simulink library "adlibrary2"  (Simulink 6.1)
undefined symbols (not defined in the file or in its folder): adlibrary2, ADM, Bit, Black, Box, d2sram_config, DDR, ddr32_config, ddr32xp_config, Generation, II, Inactive, Location, Lower, SDRAM, Simulation, Subsystem, Width, xbsIndex_r3, XPL, XRC, XRM, zbt32_config, zbt64_config, zbtXRC4_config
libraries: xbsIndex_r3 x786
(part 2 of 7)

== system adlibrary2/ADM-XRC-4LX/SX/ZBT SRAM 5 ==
  d : Inport  Port=1  LatchInput=off
  a : Inport  Port=2  LatchInput=off
  w : Inport  Port=3  LatchInput=off
  r : Inport  Port=4  LatchInput=off
  be : Inport  Port=5  LatchInput=off
  adlocb_in : Inport  Port=6  LatchInput=off
  Constant : xbsIndex_r3/Constant  const=0  equ=P=C  arith_type=Unsigned  n_bits=34  bin_pt=0  opselect=C  inp2=PCIN>>17  opr=+  inp1=P  carry=CIN  iostate=0  explicit_period=on  period=1  dbl_ovrd=off
  Convert : xbsIndex_r3/Convert  arith_type=Unsigned  n_bits=34  bin_pt=0  quantization=Truncate  overflow=Wrap  latency=0  explicit_period=on  period=1  dbl_ovrd=off  show_param=off  inserted_by_tool=off  pipeline=off
  Simulation Multiplexer : xbsIndex_r3/Simulation Multiplexer  sim_sel=1  hw_sel=2
  Simulation Multiplexer1 : xbsIndex_r3/Simulation Multiplexer  sim_sel=1  hw_sel=2
  Simulation Multiplexer2 : xbsIndex_r3/Simulation Multiplexer  sim_sel=1  hw_sel=2
  ZBT SRAM 32Bit Generation : Subsystem
  ZBT SRAM 32Bit Simulation : Subsystem
  q : Outport
  qv : Outport  Port=2
  adlocb_out : Outport  Port=3
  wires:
  r/1 -> ZBT SRAM 32Bit Generation/4(r), ZBT SRAM 32Bit Simulation/4(r)
  w/1 -> ZBT SRAM 32Bit Generation/3(w), ZBT SRAM 32Bit Simulation/3(w)
  a/1 -> ZBT SRAM 32Bit Generation/2(a), ZBT SRAM 32Bit Simulation/2(a)
  d/1 -> ZBT SRAM 32Bit Generation/1(d), ZBT SRAM 32Bit Simulation/1(d)
  ZBT SRAM 32Bit Simulation/2(qv) -> Simulation Multiplexer1/1
  ZBT SRAM 32Bit Simulation/1(q) -> Simulation Multiplexer/1
  ZBT SRAM 32Bit Generation/1(q) -> Simulation Multiplexer/2
  ZBT SRAM 32Bit Generation/2(qv) -> Simulation Multiplexer1/2
  Simulation Multiplexer1/1 -> qv/1
  Simulation Multiplexer/1 -> q/1
  be/1 -> ZBT SRAM 32Bit Simulation/5(be), ZBT SRAM 32Bit Generation/5(be)
  Simulation Multiplexer2/1 -> adlocb_out/1
  ZBT SRAM 32Bit Generation/3(adlocb_out) -> Convert/1
  adlocb_in/1 -> ZBT SRAM 32Bit Generation/6(adlocb_in)
  Constant/1 -> Simulation Multiplexer2/1
  Convert/1 -> Simulation Multiplexer2/2

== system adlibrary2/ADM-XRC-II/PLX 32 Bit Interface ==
  Data_Read : Inport  Port=1  LatchInput=off
  Ack : Inport  Port=2  LatchInput=off
  Status : Inport  Port=3  LatchInput=off
  Read IFIFO : Inport  Port=4  LatchInput=off
  Write OFIFO : Inport  Port=5  LatchInput=off
  OFIFO_Data : Inport  Port=6  LatchInput=off
  ADLOCB_IN : Inport  Port=7  LatchInput=off
  Constant : xbsIndex_r3/Constant  const=0  equ=P=C  arith_type=Unsigned  n_bits=34  bin_pt=0  opselect=C  inp2=PCIN>>17  opr=+  inp1=P  carry=CIN  iostate=0  explicit_period=on  period=1  dbl_ovrd=off
  Convert : xbsIndex_r3/Convert  arith_type=Unsigned  n_bits=34  bin_pt=0  quantization=Truncate  overflow=Wrap  latency=0  explicit_period=on  period=1  dbl_ovrd=off  show_param=off  inserted_by_tool=off  pipeline=off
  PLX 32Bit Generation : Subsystem
  PLX 32Bit Simulation : Subsystem  mask{program=program, clock_ratio=clock_ratio}
      mask prompts: program "Local Bus Script Program"; clock_ratio "Clock Ratio"
  Simulation Multiplexer{,1..9} (10 alike) : xbsIndex_r3/Simulation Multiplexer  sim_sel=1  hw_sel=2
  Data_Write : Outport
  Addr : Outport  Port=2
  BE : Outport  Port=3
  Write : Outport  Port=4
  Read : Outport  Port=5
  Control : Outport  Port=6
  IFIFO_Data : Outport  Port=7
  IFIFO_Empty : Outport  Port=8
  OFIFO_Full : Outport  Port=9
  ADLOCB_OUT : Outport  Port=10
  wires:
  Data_Read/1 -> PLX 32Bit Generation/1(Data_Read), PLX 32Bit Simulation/1(Data_Read)
  Ack/1 -> PLX 32Bit Generation/2(Ack), PLX 32Bit Simulation/2(Ack)
  Status/1 -> PLX 32Bit Generation/3(Status), PLX 32Bit Simulation/3(Status)
  Read IFIFO/1 -> PLX 32Bit Generation/4(Read IFIFO), PLX 32Bit Simulation/4(Read IFIFO)
  Write OFIFO/1 -> PLX 32Bit Generation/5(Write OFIFO), PLX 32Bit Simulation/5(Write OFIFO)
  OFIFO_Data/1 -> PLX 32Bit Generation/6(OFIFO_Data), PLX 32Bit Simulation/6(OFIFO_Data)
  Simulation Multiplexer/1 -> Data_Write/1
  Simulation Multiplexer1/1 -> Addr/1
  Simulation Multiplexer2/1 -> Write/1
  Simulation Multiplexer3/1 -> Read/1
  Simulation Multiplexer4/1 -> Control/1
  Simulation Multiplexer5/1 -> IFIFO_Data/1
  Simulation Multiplexer6/1 -> IFIFO_Empty/1
  Simulation Multiplexer7/1 -> OFIFO_Full/1
  PLX 32Bit Generation/9(OFIFO_Full) -> Simulation Multiplexer7/2
  PLX 32Bit Generation/8(IFIFO_Empty) -> Simulation Multiplexer6/2
  PLX 32Bit Generation/7(IFIFO_Data) -> Simulation Multiplexer5/2
  PLX 32Bit Generation/6(Control) -> Simulation Multiplexer4/2
  PLX 32Bit Generation/5(Read) -> Simulation Multiplexer3/2
  PLX 32Bit Generation/4(Write) -> Simulation Multiplexer2/2
  PLX 32Bit Generation/2(Addr) -> Simulation Multiplexer1/2
  PLX 32Bit Generation/1(Data_Write) -> Simulation Multiplexer/2
  PLX 32Bit Simulation/1(Data_Write) -> Simulation Multiplexer/1
  PLX 32Bit Simulation/2(Addr) -> Simulation Multiplexer1/1
  PLX 32Bit Simulation/4(Write) -> Simulation Multiplexer2/1
  PLX 32Bit Simulation/5(Read) -> Simulation Multiplexer3/1
  PLX 32Bit Simulation/6(Control) -> Simulation Multiplexer4/1
  PLX 32Bit Simulation/7(IFIFO_Data) -> Simulation Multiplexer5/1
  PLX 32Bit Simulation/8(IFIFO_Empty) -> Simulation Multiplexer6/1
  PLX 32Bit Simulation/9(OFIFO_Full) -> Simulation Multiplexer7/1
  Simulation Multiplexer8/1 -> BE/1
  PLX 32Bit Generation/3(BE) -> Simulation Multiplexer8/2
  PLX 32Bit Simulation/3(BE) -> Simulation Multiplexer8/1
  Simulation Multiplexer9/1 -> ADLOCB_OUT/1
  PLX 32Bit Generation/10(ADLOCB_OUT) -> Convert/1
  ADLOCB_IN/1 -> PLX 32Bit Generation/7(ADLOCB_IN)
  Constant/1 -> Simulation Multiplexer9/1
  Convert/1 -> Simulation Multiplexer9/2

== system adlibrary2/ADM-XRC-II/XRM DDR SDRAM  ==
  cache_data_in : Inport  Port=1  LatchInput=off
  cache_addr : Inport  Port=2  LatchInput=off
  cache_write : Inport  Port=3  LatchInput=off
  ddr_page : Inport  Port=4  LatchInput=off
  ddr_addr : Inport  Port=5  LatchInput=off
  ddr_read : Inport  Port=6  LatchInput=off
  ddr_write : Inport  Port=7  LatchInput=off
  DDR SDRAM 64Bit Generation : Subsystem
  DDR SDRAM 64bit Simulation : Subsystem  mask{memsize=memsize}
      mask prompts: memsize "Simulation Ram Size (Mb)"
  Simulation Multiplexer : xbsIndex_r3/Simulation Multiplexer  sim_sel=1  hw_sel=2
  Simulation Multiplexer1 : xbsIndex_r3/Simulation Multiplexer  sim_sel=1  hw_sel=2
  Terminator1 : Terminator
  cache_data_out : Outport
  ddr_busy : Outport  Port=2
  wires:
  cache_data_in/1 -> DDR SDRAM 64bit Simulation/1(cache_data_in), DDR SDRAM 64Bit Generation/1(cache_data_in)
  cache_addr/1 -> DDR SDRAM 64bit Simulation/2(cache_addr), DDR SDRAM 64Bit Generation/2(cache_addr)
  cache_write/1 -> DDR SDRAM 64bit Simulation/3(cache_write), DDR SDRAM 64Bit Generation/3(cache_write)
  ddr_page/1 -> DDR SDRAM 64bit Simulation/4(ddr_page), DDR SDRAM 64Bit Generation/4(ddr_page)
  ddr_addr/1 -> DDR SDRAM 64bit Simulation/5(ddr_addr), DDR SDRAM 64Bit Generation/5(ddr_addr)
  ddr_read/1 -> DDR SDRAM 64Bit Generation/6(ddr_read), DDR SDRAM 64bit Simulation/6(ddr_read)
  ddr_write/1 -> DDR SDRAM 64Bit Generation/7(ddr_write), DDR SDRAM 64bit Simulation/7(ddr_write)
  Simulation Multiplexer/1 -> cache_data_out/1
  Simulation Multiplexer1/1 -> ddr_busy/1
  DDR SDRAM 64bit Simulation/3(ddr_status) -> Terminator1/1
  DDR SDRAM 64bit Simulation/2(ddr_busy) -> Simulation Multiplexer1/1
  DDR SDRAM 64bit Simulation/1(cache_data_out) -> Simulation Multiplexer/1
  DDR SDRAM 64Bit Generation/1(cache_data_out) -> Simulation Multiplexer/2
  DDR SDRAM 64Bit Generation/2(ddr_busy) -> Simulation Multiplexer1/2

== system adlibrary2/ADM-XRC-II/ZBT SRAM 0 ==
  d : Inport  Port=1  LatchInput=off
  a : Inport  Port=2  LatchInput=off
  w : Inport  Port=3  LatchInput=off
  r : Inport  Port=4  LatchInput=off
  be : Inport  Port=5  LatchInput=off
  adlocb_in : Inport  Port=6  LatchInput=off
  Constant : xbsIndex_r3/Constant  const=0  equ=P=C  arith_type=Unsigned  n_bits=34  bin_pt=0  opselect=C  inp2=PCIN>>17  opr=+  inp1=P  carry=CIN  iostate=0  explicit_period=on  period=1  dbl_ovrd=off
  Simulation Multiplexer : xbsIndex_r3/Simulation Multiplexer  sim_sel=1  hw_sel=2
  Simulation Multiplexer1 : xbsIndex_r3/Simulation Multiplexer  sim_sel=1  hw_sel=2
  Simulation Multiplexer2 : xbsIndex_r3/Simulation Multiplexer  sim_sel=1  hw_sel=2
  ZBT SRAM 32Bit Generation : Subsystem
  ZBT SRAM 32Bit Simulation : Subsystem
  q : Outport
  qv : Outport  Port=2
  adlocb_out : Outport  Port=3
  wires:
  r/1 -> ZBT SRAM 32Bit Generation/4(r), ZBT SRAM 32Bit Simulation/4(r)
  w/1 -> ZBT SRAM 32Bit Generation/3(w), ZBT SRAM 32Bit Simulation/3(w)
  a/1 -> ZBT SRAM 32Bit Generation/2(a), ZBT SRAM 32Bit Simulation/2(a)
  d/1 -> ZBT SRAM 32Bit Generation/1(d), ZBT SRAM 32Bit Simulation/1(d)
  ZBT SRAM 32Bit Simulation/2(qv) -> Simulation Multiplexer1/1
  ZBT SRAM 32Bit Simulation/1(q) -> Simulation Multiplexer/1
  ZBT SRAM 32Bit Generation/1(q) -> Simulation Multiplexer/2
  ZBT SRAM 32Bit Generation/2(qv) -> Simulation Multiplexer1/2
  Simulation Multiplexer1/1 -> qv/1
  Simulation Multiplexer/1 -> q/1
  be/1 -> ZBT SRAM 32Bit Simulation/5(be), ZBT SRAM 32Bit Generation/5(be)
  Simulation Multiplexer2/1 -> adlocb_out/1
  ZBT SRAM 32Bit Generation/3(adlocb_out) -> Simulation Multiplexer2/2
  adlocb_in/1 -> ZBT SRAM 32Bit Generation/6(adlocb_in)
  Constant/1 -> Simulation Multiplexer2/1

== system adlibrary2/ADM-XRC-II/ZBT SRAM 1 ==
  d : Inport  Port=1  LatchInput=off
  a : Inport  Port=2  LatchInput=off
  w : Inport  Port=3  LatchInput=off
  r : Inport  Port=4  LatchInput=off
  be : Inport  Port=5  LatchInput=off
  adlocb_in : Inport  Port=6  LatchInput=off
  Constant : xbsIndex_r3/Constant  const=0  equ=P=C  arith_type=Unsigned  n_bits=34  bin_pt=0  opselect=C  inp2=PCIN>>17  opr=+  inp1=P  carry=CIN  iostate=0  explicit_period=on  period=1  dbl_ovrd=off
  Convert : xbsIndex_r3/Convert  arith_type=Unsigned  n_bits=34  bin_pt=0  quantization=Truncate  overflow=Wrap  latency=0  explicit_period=on  period=1  dbl_ovrd=off  show_param=off  inserted_by_tool=off  pipeline=off
  Simulation Multiplexer : xbsIndex_r3/Simulation Multiplexer  sim_sel=1  hw_sel=2
  Simulation Multiplexer1 : xbsIndex_r3/Simulation Multiplexer  sim_sel=1  hw_sel=2
  Simulation Multiplexer2 : xbsIndex_r3/Simulation Multiplexer  sim_sel=1  hw_sel=2
  ZBT SRAM 32Bit Generation : Subsystem
  ZBT SRAM 32Bit Simulation : Subsystem
  q : Outport
  qv : Outport  Port=2
  adlocb_out : Outport  Port=3
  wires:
  Constant/1 -> Simulation Multiplexer2/1
  adlocb_in/1 -> ZBT SRAM 32Bit Generation/6(adlocb_in)
  ZBT SRAM 32Bit Generation/3(adlocb_out) -> Convert/1
  Simulation Multiplexer2/1 -> adlocb_out/1
  be/1 -> ZBT SRAM 32Bit Generation/5(be), ZBT SRAM 32Bit Simulation/5(be)
  Simulation Multiplexer/1 -> q/1
  Simulation Multiplexer1/1 -> qv/1
  ZBT SRAM 32Bit Generation/2(qv) -> Simulation Multiplexer1/2
  ZBT SRAM 32Bit Generation/1(q) -> Simulation Multiplexer/2
  ZBT SRAM 32Bit Simulation/1(q) -> Simulation Multiplexer/1
  ZBT SRAM 32Bit Simulation/2(qv) -> Simulation Multiplexer1/1
  d/1 -> ZBT SRAM 32Bit Simulation/1(d), ZBT SRAM 32Bit Generation/1(d)
  a/1 -> ZBT SRAM 32Bit Simulation/2(a), ZBT SRAM 32Bit Generation/2(a)
  w/1 -> ZBT SRAM 32Bit Simulation/3(w), ZBT SRAM 32Bit Generation/3(w)
  r/1 -> ZBT SRAM 32Bit Simulation/4(r), ZBT SRAM 32Bit Generation/4(r)
  Convert/1 -> Simulation Multiplexer2/2

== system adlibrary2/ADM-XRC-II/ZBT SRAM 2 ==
  d : Inport  Port=1  LatchInput=off
  a : Inport  Port=2  LatchInput=off
  w : Inport  Port=3  LatchInput=off
  r : Inport  Port=4  LatchInput=off
  be : Inport  Port=5  LatchInput=off
  adlocb_in : Inport  Port=6  LatchInput=off
  Constant : xbsIndex_r3/Constant  const=0  equ=P=C  arith_type=Unsigned  n_bits=34  bin_pt=0  opselect=C  inp2=PCIN>>17  opr=+  inp1=P  carry=CIN  iostate=0  explicit_period=on  period=1  dbl_ovrd=off
  Convert : xbsIndex_r3/Convert  arith_type=Unsigned  n_bits=34  bin_pt=0  quantization=Truncate  overflow=Wrap  latency=0  explicit_period=on  period=1  dbl_ovrd=off  show_param=off  inserted_by_tool=off  pipeline=off
  Simulation Multiplexer : xbsIndex_r3/Simulation Multiplexer  sim_sel=1  hw_sel=2
  Simulation Multiplexer1 : xbsIndex_r3/Simulation Multiplexer  sim_sel=1  hw_sel=2
  Simulation Multiplexer2 : xbsIndex_r3/Simulation Multiplexer  sim_sel=1  hw_sel=2
  ZBT SRAM 32Bit Generation : Subsystem
  ZBT SRAM 32Bit Simulation : Subsystem
  q : Outport
  qv : Outport  Port=2
  adlocb_out : Outport  Port=3
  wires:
  Constant/1 -> Simulation Multiplexer2/1
  adlocb_in/1 -> ZBT SRAM 32Bit Generation/6(adlocb_in)
  ZBT SRAM 32Bit Generation/3(adlocb_out) -> Convert/1
  Simulation Multiplexer2/1 -> adlocb_out/1
  be/1 -> ZBT SRAM 32Bit Generation/5(be), ZBT SRAM 32Bit Simulation/5(be)
  Simulation Multiplexer/1 -> q/1
  Simulation Multiplexer1/1 -> qv/1
  ZBT SRAM 32Bit Generation/2(qv) -> Simulation Multiplexer1/2
  ZBT SRAM 32Bit Generation/1(q) -> Simulation Multiplexer/2
  ZBT SRAM 32Bit Simulation/1(q) -> Simulation Multiplexer/1
  ZBT SRAM 32Bit Simulation/2(qv) -> Simulation Multiplexer1/1
  d/1 -> ZBT SRAM 32Bit Simulation/1(d), ZBT SRAM 32Bit Generation/1(d)
  a/1 -> ZBT SRAM 32Bit Simulation/2(a), ZBT SRAM 32Bit Generation/2(a)
  w/1 -> ZBT SRAM 32Bit Simulation/3(w), ZBT SRAM 32Bit Generation/3(w)
  r/1 -> ZBT SRAM 32Bit Simulation/4(r), ZBT SRAM 32Bit Generation/4(r)
  Convert/1 -> Simulation Multiplexer2/2

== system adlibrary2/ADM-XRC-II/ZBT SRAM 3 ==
  d : Inport  Port=1  LatchInput=off
  a : Inport  Port=2  LatchInput=off
  w : Inport  Port=3  LatchInput=off
  r : Inport  Port=4  LatchInput=off
  be : Inport  Port=5  LatchInput=off
  adlocb_in : Inport  Port=6  LatchInput=off
  Constant : xbsIndex_r3/Constant  const=0  equ=P=C  arith_type=Unsigned  n_bits=34  bin_pt=0  opselect=C  inp2=PCIN>>17  opr=+  inp1=P  carry=CIN  iostate=0  explicit_period=on  period=1  dbl_ovrd=off
  Convert : xbsIndex_r3/Convert  arith_type=Unsigned  n_bits=34  bin_pt=0  quantization=Truncate  overflow=Wrap  latency=0  explicit_period=on  period=1  dbl_ovrd=off  show_param=off  inserted_by_tool=off  pipeline=off
  Simulation Multiplexer : xbsIndex_r3/Simulation Multiplexer  sim_sel=1  hw_sel=2
  Simulation Multiplexer1 : xbsIndex_r3/Simulation Multiplexer  sim_sel=1  hw_sel=2
  Simulation Multiplexer2 : xbsIndex_r3/Simulation Multiplexer  sim_sel=1  hw_sel=2
  ZBT SRAM 32Bit Generation : Subsystem
  ZBT SRAM 32Bit Simulation : Subsystem
  q : Outport
  qv : Outport  Port=2
  adlocb_out : Outport  Port=3
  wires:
  r/1 -> ZBT SRAM 32Bit Generation/4(r), ZBT SRAM 32Bit Simulation/4(r)
  w/1 -> ZBT SRAM 32Bit Generation/3(w), ZBT SRAM 32Bit Simulation/3(w)
  a/1 -> ZBT SRAM 32Bit Generation/2(a), ZBT SRAM 32Bit Simulation/2(a)
  d/1 -> ZBT SRAM 32Bit Generation/1(d), ZBT SRAM 32Bit Simulation/1(d)
  ZBT SRAM 32Bit Simulation/2(qv) -> Simulation Multiplexer1/1
  ZBT SRAM 32Bit Simulation/1(q) -> Simulation Multiplexer/1
  ZBT SRAM 32Bit Generation/1(q) -> Simulation Multiplexer/2
  ZBT SRAM 32Bit Generation/2(qv) -> Simulation Multiplexer1/2
  Simulation Multiplexer1/1 -> qv/1
  Simulation Multiplexer/1 -> q/1
  be/1 -> ZBT SRAM 32Bit Simulation/5(be), ZBT SRAM 32Bit Generation/5(be)
  Simulation Multiplexer2/1 -> adlocb_out/1
  ZBT SRAM 32Bit Generation/3(adlocb_out) -> Convert/1
  adlocb_in/1 -> ZBT SRAM 32Bit Generation/6(adlocb_in)
  Constant/1 -> Simulation Multiplexer2/1
  Convert/1 -> Simulation Multiplexer2/2

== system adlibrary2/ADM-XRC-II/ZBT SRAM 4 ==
  d : Inport  Port=1  LatchInput=off
  a : Inport  Port=2  LatchInput=off
  w : Inport  Port=3  LatchInput=off
  r : Inport  Port=4  LatchInput=off
  be : Inport  Port=5  LatchInput=off
  adlocb_in : Inport  Port=6  LatchInput=off
  Constant : xbsIndex_r3/Constant  const=0  equ=P=C  arith_type=Unsigned  n_bits=34  bin_pt=0  opselect=C  inp2=PCIN>>17  opr=+  inp1=P  carry=CIN  iostate=0  explicit_period=on  period=1  dbl_ovrd=off
  Convert : xbsIndex_r3/Convert  arith_type=Unsigned  n_bits=34  bin_pt=0  quantization=Truncate  overflow=Wrap  latency=0  explicit_period=on  period=1  dbl_ovrd=off  show_param=off  inserted_by_tool=off  pipeline=off
  Simulation Multiplexer : xbsIndex_r3/Simulation Multiplexer  sim_sel=1  hw_sel=2
  Simulation Multiplexer1 : xbsIndex_r3/Simulation Multiplexer  sim_sel=1  hw_sel=2
  Simulation Multiplexer2 : xbsIndex_r3/Simulation Multiplexer  sim_sel=1  hw_sel=2
  ZBT SRAM 32Bit Generation : Subsystem
  ZBT SRAM 32Bit Simulation : Subsystem
  q : Outport
  qv : Outport  Port=2
  adlocb_out : Outport  Port=3
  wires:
  Constant/1 -> Simulation Multiplexer2/1
  adlocb_in/1 -> ZBT SRAM 32Bit Generation/6(adlocb_in)
  ZBT SRAM 32Bit Generation/3(adlocb_out) -> Convert/1
  Simulation Multiplexer2/1 -> adlocb_out/1
  be/1 -> ZBT SRAM 32Bit Generation/5(be), ZBT SRAM 32Bit Simulation/5(be)
  Simulation Multiplexer/1 -> q/1
  Simulation Multiplexer1/1 -> qv/1
  ZBT SRAM 32Bit Generation/2(qv) -> Simulation Multiplexer1/2
  ZBT SRAM 32Bit Generation/1(q) -> Simulation Multiplexer/2
  ZBT SRAM 32Bit Simulation/1(q) -> Simulation Multiplexer/1
  ZBT SRAM 32Bit Simulation/2(qv) -> Simulation Multiplexer1/1
  d/1 -> ZBT SRAM 32Bit Simulation/1(d), ZBT SRAM 32Bit Generation/1(d)
  a/1 -> ZBT SRAM 32Bit Simulation/2(a), ZBT SRAM 32Bit Generation/2(a)
  w/1 -> ZBT SRAM 32Bit Simulation/3(w), ZBT SRAM 32Bit Generation/3(w)
  r/1 -> ZBT SRAM 32Bit Simulation/4(r), ZBT SRAM 32Bit Generation/4(r)
  Convert/1 -> Simulation Multiplexer2/2

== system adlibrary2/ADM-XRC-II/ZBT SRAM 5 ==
  d : Inport  Port=1  LatchInput=off
  a : Inport  Port=2  LatchInput=off
  w : Inport  Port=3  LatchInput=off
  r : Inport  Port=4  LatchInput=off
  be : Inport  Port=5  LatchInput=off
  adlocb_in : Inport  Port=6  LatchInput=off
  Constant : xbsIndex_r3/Constant  const=0  equ=P=C  arith_type=Unsigned  n_bits=34  bin_pt=0  opselect=C  inp2=PCIN>>17  opr=+  inp1=P  carry=CIN  iostate=0  explicit_period=on  period=1  dbl_ovrd=off
  Convert : xbsIndex_r3/Convert  arith_type=Unsigned  n_bits=34  bin_pt=0  quantization=Truncate  overflow=Wrap  latency=0  explicit_period=on  period=1  dbl_ovrd=off  show_param=off  inserted_by_tool=off  pipeline=off
  Simulation Multiplexer : xbsIndex_r3/Simulation Multiplexer  sim_sel=1  hw_sel=2
  Simulation Multiplexer1 : xbsIndex_r3/Simulation Multiplexer  sim_sel=1  hw_sel=2
  Simulation Multiplexer2 : xbsIndex_r3/Simulation Multiplexer  sim_sel=1  hw_sel=2
  ZBT SRAM 32Bit Generation : Subsystem
  ZBT SRAM 32Bit Simulation : Subsystem
  q : Outport
  qv : Outport  Port=2
  adlocb_out : Outport  Port=3
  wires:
  r/1 -> ZBT SRAM 32Bit Generation/4(r), ZBT SRAM 32Bit Simulation/4(r)
  w/1 -> ZBT SRAM 32Bit Generation/3(w), ZBT SRAM 32Bit Simulation/3(w)
  a/1 -> ZBT SRAM 32Bit Generation/2(a), ZBT SRAM 32Bit Simulation/2(a)
  d/1 -> ZBT SRAM 32Bit Generation/1(d), ZBT SRAM 32Bit Simulation/1(d)
  ZBT SRAM 32Bit Simulation/2(qv) -> Simulation Multiplexer1/1
  ZBT SRAM 32Bit Simulation/1(q) -> Simulation Multiplexer/1
  ZBT SRAM 32Bit Generation/1(q) -> Simulation Multiplexer/2
  ZBT SRAM 32Bit Generation/2(qv) -> Simulation Multiplexer1/2
  Simulation Multiplexer1/1 -> qv/1
  Simulation Multiplexer/1 -> q/1
  be/1 -> ZBT SRAM 32Bit Simulation/5(be), ZBT SRAM 32Bit Generation/5(be)
  Simulation Multiplexer2/1 -> adlocb_out/1
  ZBT SRAM 32Bit Generation/3(adlocb_out) -> Convert/1
  adlocb_in/1 -> ZBT SRAM 32Bit Generation/6(adlocb_in)
  Constant/1 -> Simulation Multiplexer2/1
  Convert/1 -> Simulation Multiplexer2/2

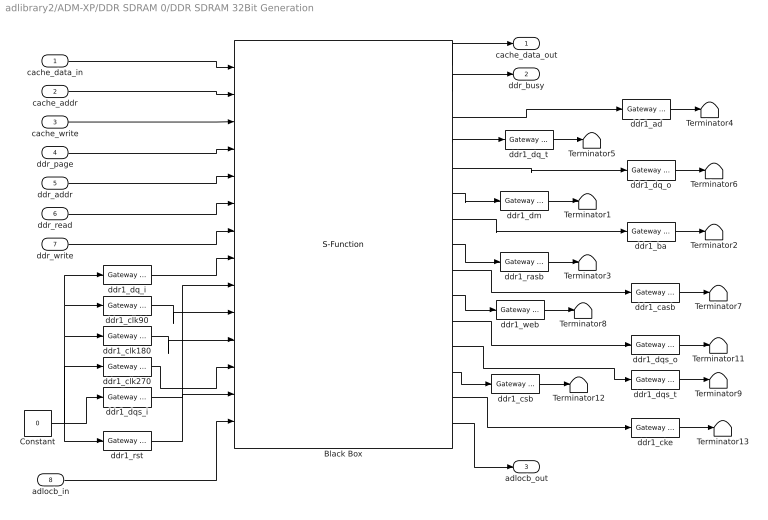
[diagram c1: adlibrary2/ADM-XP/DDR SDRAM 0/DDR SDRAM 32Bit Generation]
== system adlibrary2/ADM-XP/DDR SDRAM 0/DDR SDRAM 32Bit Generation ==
  cache_data_in : Inport  Port=1  LatchInput=off
  cache_addr : Inport  Port=2  LatchInput=off
  cache_write : Inport  Port=3  LatchInput=off
  ddr_page : Inport  Port=4  LatchInput=off
  ddr_addr : Inport  Port=5  LatchInput=off
  ddr_read : Inport  Port=6  LatchInput=off
  ddr_write : Inport  Port=7  LatchInput=off
  adlocb_in : Inport  Port=8  LatchInput=off
  Black Box : S-Function  AncestorBlock=xbsIndex_r3/Black Box  FunctionName=xlblackbox2  Parameters=sfcn_mwsv__  mask(Xilinx Blackbox Block){init_code=ddr32xp_config, sim_method=Inactive, engine_block=, show_param=on, xl_area=[375, 550, 2, 337, 9, 0, 0], xl_use_area=on, adlocb_devid=4, ddr_size=64}
      mask prompts: init_code "Block Configuration M-Function"; sim_method "Simulation Mode"; engine_block "HDL Co-Simulator To Use  (specify helper block by name)"; show_param "---------------------- Show Implementation Parameters -----------------------------------------------------------------------------------"; xl_area "FPGA Area [Slices, FFs, BRAMs, LUTs, IOBs, Emb. Mults, TBUFs]"; xl_use_area "Use Area Above For Estimation"; adlocb_devid "ADLOCB DEV ID"; ddr_size "DDR BANK SIZE(MB)"
      mask help: Incorporates black box HDL and simulation model into a System Generator design. You must supply a Black Box with certain information about the HDL component you would like to bring into System Generator. This information is provided through a Matlab function. When "Simulation Mode" is set to "Inactive," you will typically want to provide a separate simulation model by using a Simulation Multiplexer. When "Simulation Mode" is set to "Use HDL Co-Simulation", you must include a ModelSim block in the design.
      mask init:
      | [designRoot, family, part, speed, package, simulinkPeriod, sysclkPeriod, dbl_ovrd, trimVbit] = xlSysgenSettings(gcb,0,0);
      | 
      | [bg,fg] = xlcmap('XBlock');
      | iPos = get_param(gcb,'Position');
      | iWidth=iPos(3)-iPos(1); iHeight=iPos(4)-iPos(2);
      | iCx=iWidth/2;
      | iCy=iHeight/2;
      | [logoX, logoY] = xlogo(iPos);
      | zstr='z'; zpstr='-1';
      | zstrx = iCx-3; if (zstrx<16) zstr='';zpstr=''; end
      | zstry = iCy;
      | 
      | precision0 = 1;
      | latency = 0;
      | dblOvrd = 0;
      | 
      | mdlPath = xlGetMdlDir(bdroot);
      | 
      | refBlk = get_param(gcb,'referenceBlock');
      | if (isempty(refBlk) | strncmp(refBlk,'xbsIndex',8))
      | 	srcPath = mdlPath;
      | else
      | 	srcPath = xlPathToReference;
      | 	if (isempty(srcPath))
      | 		srcPath = mdlPath;
      | 	end
      | end
      | 
      | if (sim_method==2)
      | 	validEngineBlock = 0;
      | 	try
      | 	  engineBlock = xlBlockNameRelPath(get_param(gcb,'Parent'),engine_block);
      | 	catch
      | 	  engineBlock = '//';
      | 	end
      | 	try 
      | 	  engineWorkDir = get_param(engineBlock,'dir');
      | 	  validEngineBlock = 1;
      | 	catch
      | 	end
      | end
      | 
      | % just pass everything to s-function
      | sfcn_mwsv__ = get_param(gcb, 'MaskWSVariables');
      | 
      | plabel = xlbbPortLabelStruct(gcb,init_code,mdlPath);
  Constant : Constant  Value=0
  Terminator{1..9,11..13} (12 alike) : Terminator
  ddr1_ad : xbsIndex_r3/Gateway Out  output_type=Double  nbits=8  bin_pt=6  arith_type=Boolean  quantization=Truncate  overflow=Wrap  hdl_port=on  timing_constraint=None  locs_specified=off  LOCs={}  needs_fixed_name=off  show_param=off
  ddr1_ba : xbsIndex_r3/Gateway Out  output_type=Double  nbits=8  bin_pt=6  arith_type=Boolean  quantization=Truncate  overflow=Wrap  hdl_port=on  timing_constraint=None  locs_specified=off  LOCs={}  needs_fixed_name=off  show_param=off
  ddr1_casb : xbsIndex_r3/Gateway Out  output_type=Double  nbits=8  bin_pt=6  arith_type=Boolean  quantization=Truncate  overflow=Wrap  hdl_port=on  timing_constraint=None  locs_specified=off  LOCs={}  needs_fixed_name=off  show_param=off
  ddr1_cke : xbsIndex_r3/Gateway Out  output_type=Double  nbits=8  bin_pt=6  arith_type=Boolean  quantization=Truncate  overflow=Wrap  hdl_port=on  timing_constraint=None  locs_specified=off  LOCs={}  needs_fixed_name=off  show_param=off
  ddr1_clk180 : xbsIndex_r3/Gateway In  arith_type=Boolean  n_bits=64  bin_pt=0  quantization=Truncate  overflow=Wrap  period=1  timing_constraint=None  locs_specified=off  LOCs={}  needs_fixed_name=off  dbl_ovrd=off  show_param=off
  ddr1_clk270 : xbsIndex_r3/Gateway In  arith_type=Boolean  n_bits=64  bin_pt=0  quantization=Truncate  overflow=Wrap  period=1  timing_constraint=None  locs_specified=off  LOCs={}  needs_fixed_name=off  dbl_ovrd=off  show_param=off
  ddr1_clk90 : xbsIndex_r3/Gateway In  arith_type=Boolean  n_bits=64  bin_pt=0  quantization=Truncate  overflow=Wrap  period=1  timing_constraint=None  locs_specified=off  LOCs={}  needs_fixed_name=off  dbl_ovrd=off  show_param=off
  ddr1_csb : xbsIndex_r3/Gateway Out  output_type=Double  nbits=8  bin_pt=6  arith_type=Boolean  quantization=Truncate  overflow=Wrap  hdl_port=on  timing_constraint=None  locs_specified=off  LOCs={}  needs_fixed_name=off  show_param=off
  ddr1_dm : xbsIndex_r3/Gateway Out  output_type=Double  nbits=8  bin_pt=6  arith_type=Boolean  quantization=Truncate  overflow=Wrap  hdl_port=on  timing_constraint=None  locs_specified=off  LOCs={}  needs_fixed_name=off  show_param=off
  ddr1_dq_i : xbsIndex_r3/Gateway In  arith_type=Unsigned  n_bits=32  bin_pt=0  quantization=Truncate  overflow=Wrap  period=1  timing_constraint=None  locs_specified=off  LOCs={}  needs_fixed_name=off  dbl_ovrd=off  show_param=off
  ddr1_dq_o : xbsIndex_r3/Gateway Out  output_type=Double  nbits=8  bin_pt=6  arith_type=Boolean  quantization=Truncate  overflow=Wrap  hdl_port=on  timing_constraint=None  locs_specified=off  LOCs={}  needs_fixed_name=off  show_param=off
  ddr1_dq_t : xbsIndex_r3/Gateway Out  output_type=Double  nbits=8  bin_pt=6  arith_type=Boolean  quantization=Truncate  overflow=Wrap  hdl_port=on  timing_constraint=None  locs_specified=off  LOCs={}  needs_fixed_name=off  show_param=off
  ddr1_dqs_i : xbsIndex_r3/Gateway In  arith_type=Unsigned  n_bits=4  bin_pt=0  quantization=Truncate  overflow=Wrap  period=1  timing_constraint=None  locs_specified=off  LOCs={}  needs_fixed_name=off  dbl_ovrd=off  show_param=off
  ddr1_dqs_o : xbsIndex_r3/Gateway Out  output_type=Double  nbits=8  bin_pt=6  arith_type=Boolean  quantization=Truncate  overflow=Wrap  hdl_port=on  timing_constraint=None  locs_specified=off  LOCs={}  needs_fixed_name=off  show_param=off
  ddr1_dqs_t : xbsIndex_r3/Gateway Out  output_type=Double  nbits=8  bin_pt=6  arith_type=Boolean  quantization=Truncate  overflow=Wrap  hdl_port=on  timing_constraint=None  locs_specified=off  LOCs={}  needs_fixed_name=off  show_param=off
  ddr1_rasb : xbsIndex_r3/Gateway Out  output_type=Double  nbits=8  bin_pt=6  arith_type=Boolean  quantization=Truncate  overflow=Wrap  hdl_port=on  timing_constraint=None  locs_specified=off  LOCs={}  needs_fixed_name=off  show_param=off
  ddr1_rst : xbsIndex_r3/Gateway In  arith_type=Boolean  n_bits=64  bin_pt=0  quantization=Truncate  overflow=Wrap  period=1  timing_constraint=None  locs_specified=off  LOCs={}  needs_fixed_name=off  dbl_ovrd=off  show_param=off
  ddr1_web : xbsIndex_r3/Gateway Out  output_type=Double  nbits=8  bin_pt=6  arith_type=Boolean  quantization=Truncate  overflow=Wrap  hdl_port=on  timing_constraint=None  locs_specified=off  LOCs={}  needs_fixed_name=off  show_param=off
  cache_data_out : Outport
  ddr_busy : Outport  Port=2
  adlocb_out : Outport  Port=3
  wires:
  ddr1_cke/1 -> Terminator13/1
  ddr1_csb/1 -> Terminator12/1
  ddr1_dqs_o/1 -> Terminator11/1
  ddr1_web/1 -> Terminator8/1
  ddr1_casb/1 -> Terminator7/1
  ddr1_rasb/1 -> Terminator3/1
  ddr1_ba/1 -> Terminator2/1
  ddr1_dm/1 -> Terminator1/1
  ddr1_dq_o/1 -> Terminator6/1
  ddr1_dq_t/1 -> Terminator5/1
  ddr1_ad/1 -> Terminator4/1
  Black Box/2 -> ddr_busy/1
  Black Box/1 -> cache_data_out/1
  ddr_write/1 -> Black Box/7
  ddr_read/1 -> Black Box/6
  ddr_addr/1 -> Black Box/5
  ddr_page/1 -> Black Box/4
  cache_write/1 -> Black Box/3
  cache_addr/1 -> Black Box/2
  cache_data_in/1 -> Black Box/1
  ddr1_dq_i/1 -> Black Box/8
  Constant/1 -> ddr1_dq_i/1, ddr1_clk90/1, ddr1_clk180/1, ddr1_clk270/1, ddr1_dqs_i/1, ddr1_rst/1
  ddr1_dqs_t/1 -> Terminator9/1
  Black Box/3 -> ddr1_ad/1
  Black Box/4 -> ddr1_dq_t/1
  Black Box/5 -> ddr1_dq_o/1
  Black Box/6 -> ddr1_dm/1
  Black Box/7 -> ddr1_ba/1
  Black Box/8 -> ddr1_rasb/1
  Black Box/9 -> ddr1_casb/1
  Black Box/10 -> ddr1_web/1
  Black Box/11 -> ddr1_dqs_o/1
  Black Box/12 -> ddr1_dqs_t/1
  Black Box/13 -> ddr1_csb/1
  Black Box/14 -> ddr1_cke/1
  Black Box/15 -> adlocb_out/1
  ddr1_dqs_i/1 -> Black Box/9
  ddr1_clk90/1 -> Black Box/10
  ddr1_clk180/1 -> Black Box/11
  ddr1_clk270/1 -> Black Box/12
  adlocb_in/1 -> Black Box/14
  ddr1_rst/1 -> Black Box/13

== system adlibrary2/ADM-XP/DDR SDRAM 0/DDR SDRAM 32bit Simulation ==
  cache_data_in : Inport  Port=1  LatchInput=off
  cache_addr : Inport  Port=2  LatchInput=off
  cache_write : Inport  Port=3  LatchInput=off
  ddr_page : Inport  Port=4  LatchInput=off
  ddr_addr : Inport  Port=5  LatchInput=off
  ddr_read : Inport  Port=6  LatchInput=off
  ddr_write : Inport  Port=7  LatchInput=off
  Disregard Subsystem : xbsIndex_r3/Disregard Subsystem  Tag=discardX
  S-Function : S-Function  FunctionName=ddr32  Parameters=memsize,0
  Subsystem : Subsystem  AncestorBlock=adlibrary2/ADM-XRC-II/XRM DDR SDRAM /DDR SDRAM 64bit Simulation/Subsystem
  Terminator13 : Terminator
  gi{0..6} (7 alike) : xbsIndex_r3/Gateway Out  output_type=Double  nbits=8  bin_pt=6  arith_type=Boolean  quantization=Truncate  overflow=Wrap  hdl_port=off  timing_constraint=None  locs_specified=off  LOCs={}  needs_fixed_name=off  show_param=off
  cache_data_out : Outport
  ddr_busy : Outport  Port=2
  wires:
  cache_data_in/1 -> gi0/1
  cache_addr/1 -> gi1/1
  cache_write/1 -> gi2/1
  ddr_page/1 -> gi3/1
  ddr_addr/1 -> gi4/1
  ddr_read/1 -> gi5/1
  ddr_write/1 -> gi6/1
  gi0/1 -> S-Function/1
  gi1/1 -> S-Function/2
  gi2/1 -> S-Function/3
  gi3/1 -> S-Function/4
  gi4/1 -> S-Function/5
  gi5/1 -> S-Function/6
  gi6/1 -> S-Function/7
  S-Function/2 -> Subsystem/2(In2)
  S-Function/1 -> Subsystem/1(In1)
  Subsystem/1(Out1) -> cache_data_out/1
  Subsystem/2(Out2) -> ddr_busy/1
  S-Function/3 -> Terminator13/1

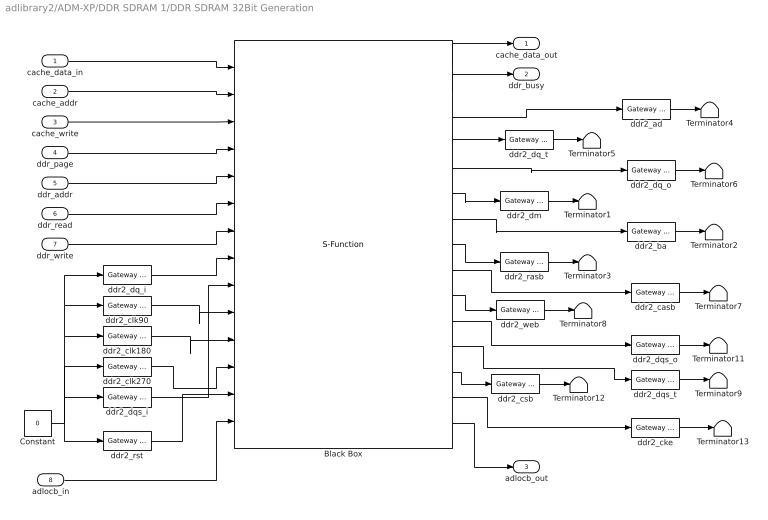
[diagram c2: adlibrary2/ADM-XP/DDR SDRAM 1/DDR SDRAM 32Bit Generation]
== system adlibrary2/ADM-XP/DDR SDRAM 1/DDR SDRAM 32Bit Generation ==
  cache_data_in : Inport  Port=1  LatchInput=off
  cache_addr : Inport  Port=2  LatchInput=off
  cache_write : Inport  Port=3  LatchInput=off
  ddr_page : Inport  Port=4  LatchInput=off
  ddr_addr : Inport  Port=5  LatchInput=off
  ddr_read : Inport  Port=6  LatchInput=off
  ddr_write : Inport  Port=7  LatchInput=off
  adlocb_in : Inport  Port=8  LatchInput=off
  Black Box : S-Function  AncestorBlock=xbsIndex_r3/Black Box  FunctionName=xlblackbox2  Parameters=sfcn_mwsv__  mask(Xilinx Blackbox Block){init_code=ddr32xp_config, sim_method=Inactive, engine_block=, show_param=on, xl_area=[375, 550, 2, 337, 9, 0, 0], xl_use_area=on, adlocb_devid=5, ddr_size=64}
      mask prompts: init_code "Block Configuration M-Function"; sim_method "Simulation Mode"; engine_block "HDL Co-Simulator To Use  (specify helper block by name)"; show_param "---------------------- Show Implementation Parameters -----------------------------------------------------------------------------------"; xl_area "FPGA Area [Slices, FFs, BRAMs, LUTs, IOBs, Emb. Mults, TBUFs]"; xl_use_area "Use Area Above For Estimation"; adlocb_devid "ADLOCB DEV ID"; ddr_size "DDR BANK SIZE(MB)"
      mask help: Incorporates black box HDL and simulation model into a System Generator design. You must supply a Black Box with certain information about the HDL component you would like to bring into System Generator. This information is provided through a Matlab function. When "Simulation Mode" is set to "Inactive," you will typically want to provide a separate simulation model by using a Simulation Multiplexer. When "Simulation Mode" is set to "Use HDL Co-Simulation", you must include a ModelSim block in the design.
      mask init:
      | [designRoot, family, part, speed, package, simulinkPeriod, sysclkPeriod, dbl_ovrd, trimVbit] = xlSysgenSettings(gcb,0,0);
      | 
      | [bg,fg] = xlcmap('XBlock');
      | iPos = get_param(gcb,'Position');
      | iWidth=iPos(3)-iPos(1); iHeight=iPos(4)-iPos(2);
      | iCx=iWidth/2;
      | iCy=iHeight/2;
      | [logoX, logoY] = xlogo(iPos);
      | zstr='z'; zpstr='-1';
      | zstrx = iCx-3; if (zstrx<16) zstr='';zpstr=''; end
      | zstry = iCy;
      | 
      | precision0 = 1;
      | latency = 0;
      | dblOvrd = 0;
      | 
      | mdlPath = xlGetMdlDir(bdroot);
      | 
      | refBlk = get_param(gcb,'referenceBlock');
      | if (isempty(refBlk) | strncmp(refBlk,'xbsIndex',8))
      | 	srcPath = mdlPath;
      | else
      | 	srcPath = xlPathToReference;
      | 	if (isempty(srcPath))
      | 		srcPath = mdlPath;
      | 	end
      | end
      | 
      | if (sim_method==2)
      | 	validEngineBlock = 0;
      | 	try
      | 	  engineBlock = xlBlockNameRelPath(get_param(gcb,'Parent'),engine_block);
      | 	catch
      | 	  engineBlock = '//';
      | 	end
      | 	try 
      | 	  engineWorkDir = get_param(engineBlock,'dir');
      | 	  validEngineBlock = 1;
      | 	catch
      | 	end
      | end
      | 
      | % just pass everything to s-function
      | sfcn_mwsv__ = get_param(gcb, 'MaskWSVariables');
      | 
      | plabel = xlbbPortLabelStruct(gcb,init_code,mdlPath);
  Constant : Constant  Value=0
  Terminator{1..9,11..13} (12 alike) : Terminator
  ddr2_ad : xbsIndex_r3/Gateway Out  output_type=Double  nbits=8  bin_pt=6  arith_type=Boolean  quantization=Truncate  overflow=Wrap  hdl_port=on  timing_constraint=None  locs_specified=off  LOCs={}  needs_fixed_name=off  show_param=off
  ddr2_ba : xbsIndex_r3/Gateway Out  output_type=Double  nbits=8  bin_pt=6  arith_type=Boolean  quantization=Truncate  overflow=Wrap  hdl_port=on  timing_constraint=None  locs_specified=off  LOCs={}  needs_fixed_name=off  show_param=off
  ddr2_casb : xbsIndex_r3/Gateway Out  output_type=Double  nbits=8  bin_pt=6  arith_type=Boolean  quantization=Truncate  overflow=Wrap  hdl_port=on  timing_constraint=None  locs_specified=off  LOCs={}  needs_fixed_name=off  show_param=off
  ddr2_cke : xbsIndex_r3/Gateway Out  output_type=Double  nbits=8  bin_pt=6  arith_type=Boolean  quantization=Truncate  overflow=Wrap  hdl_port=on  timing_constraint=None  locs_specified=off  LOCs={}  needs_fixed_name=off  show_param=off
  ddr2_clk180 : xbsIndex_r3/Gateway In  arith_type=Boolean  n_bits=64  bin_pt=0  quantization=Truncate  overflow=Wrap  period=1  timing_constraint=None  locs_specified=off  LOCs={}  needs_fixed_name=off  dbl_ovrd=off  show_param=off
  ddr2_clk270 : xbsIndex_r3/Gateway In  arith_type=Boolean  n_bits=64  bin_pt=0  quantization=Truncate  overflow=Wrap  period=1  timing_constraint=None  locs_specified=off  LOCs={}  needs_fixed_name=off  dbl_ovrd=off  show_param=off
  ddr2_clk90 : xbsIndex_r3/Gateway In  arith_type=Boolean  n_bits=64  bin_pt=0  quantization=Truncate  overflow=Wrap  period=1  timing_constraint=None  locs_specified=off  LOCs={}  needs_fixed_name=off  dbl_ovrd=off  show_param=off
  ddr2_csb : xbsIndex_r3/Gateway Out  output_type=Double  nbits=8  bin_pt=6  arith_type=Boolean  quantization=Truncate  overflow=Wrap  hdl_port=on  timing_constraint=None  locs_specified=off  LOCs={}  needs_fixed_name=off  show_param=off
  ddr2_dm : xbsIndex_r3/Gateway Out  output_type=Double  nbits=8  bin_pt=6  arith_type=Boolean  quantization=Truncate  overflow=Wrap  hdl_port=on  timing_constraint=None  locs_specified=off  LOCs={}  needs_fixed_name=off  show_param=off
  ddr2_dq_i : xbsIndex_r3/Gateway In  arith_type=Unsigned  n_bits=32  bin_pt=0  quantization=Truncate  overflow=Wrap  period=1  timing_constraint=None  locs_specified=off  LOCs={}  needs_fixed_name=off  dbl_ovrd=off  show_param=off
  ddr2_dq_o : xbsIndex_r3/Gateway Out  output_type=Double  nbits=8  bin_pt=6  arith_type=Boolean  quantization=Truncate  overflow=Wrap  hdl_port=on  timing_constraint=None  locs_specified=off  LOCs={}  needs_fixed_name=off  show_param=off
  ddr2_dq_t : xbsIndex_r3/Gateway Out  output_type=Double  nbits=8  bin_pt=6  arith_type=Boolean  quantization=Truncate  overflow=Wrap  hdl_port=on  timing_constraint=None  locs_specified=off  LOCs={}  needs_fixed_name=off  show_param=off
  ddr2_dqs_i : xbsIndex_r3/Gateway In  arith_type=Unsigned  n_bits=4  bin_pt=0  quantization=Truncate  overflow=Wrap  period=1  timing_constraint=None  locs_specified=off  LOCs={}  needs_fixed_name=off  dbl_ovrd=off  show_param=off
  ddr2_dqs_o : xbsIndex_r3/Gateway Out  output_type=Double  nbits=8  bin_pt=6  arith_type=Boolean  quantization=Truncate  overflow=Wrap  hdl_port=on  timing_constraint=None  locs_specified=off  LOCs={}  needs_fixed_name=off  show_param=off
  ddr2_dqs_t : xbsIndex_r3/Gateway Out  output_type=Double  nbits=8  bin_pt=6  arith_type=Boolean  quantization=Truncate  overflow=Wrap  hdl_port=on  timing_constraint=None  locs_specified=off  LOCs={}  needs_fixed_name=off  show_param=off
  ddr2_rasb : xbsIndex_r3/Gateway Out  output_type=Double  nbits=8  bin_pt=6  arith_type=Boolean  quantization=Truncate  overflow=Wrap  hdl_port=on  timing_constraint=None  locs_specified=off  LOCs={}  needs_fixed_name=off  show_param=off
  ddr2_rst : xbsIndex_r3/Gateway In  arith_type=Boolean  n_bits=64  bin_pt=0  quantization=Truncate  overflow=Wrap  period=1  timing_constraint=None  locs_specified=off  LOCs={}  needs_fixed_name=off  dbl_ovrd=off  show_param=off
  ddr2_web : xbsIndex_r3/Gateway Out  output_type=Double  nbits=8  bin_pt=6  arith_type=Boolean  quantization=Truncate  overflow=Wrap  hdl_port=on  timing_constraint=None  locs_specified=off  LOCs={}  needs_fixed_name=off  show_param=off
  cache_data_out : Outport
  ddr_busy : Outport  Port=2
  adlocb_out : Outport  Port=3
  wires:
  Black Box/15 -> adlocb_out/1
  Black Box/14 -> ddr2_cke/1
  Black Box/13 -> ddr2_csb/1
  Black Box/12 -> ddr2_dqs_t/1
  Black Box/11 -> ddr2_dqs_o/1
  Black Box/10 -> ddr2_web/1
  Black Box/9 -> ddr2_casb/1
  Black Box/8 -> ddr2_rasb/1
  Black Box/7 -> ddr2_ba/1
  Black Box/6 -> ddr2_dm/1
  Black Box/5 -> ddr2_dq_o/1
  Black Box/4 -> ddr2_dq_t/1
  Black Box/3 -> ddr2_ad/1
  ddr2_dqs_t/1 -> Terminator9/1
  Constant/1 -> ddr2_dqs_i/1, ddr2_clk270/1, ddr2_clk180/1, ddr2_clk90/1, ddr2_dq_i/1, ddr2_rst/1
  ddr2_dq_i/1 -> Black Box/8
  cache_data_in/1 -> Black Box/1
  cache_addr/1 -> Black Box/2
  cache_write/1 -> Black Box/3
  ddr_page/1 -> Black Box/4
  ddr_addr/1 -> Black Box/5
  ddr_read/1 -> Black Box/6
  ddr_write/1 -> Black Box/7
  Black Box/1 -> cache_data_out/1
  Black Box/2 -> ddr_busy/1
  ddr2_ad/1 -> Terminator4/1
  ddr2_dq_t/1 -> Terminator5/1
  ddr2_dq_o/1 -> Terminator6/1
  ddr2_dm/1 -> Terminator1/1
  ddr2_ba/1 -> Terminator2/1
  ddr2_rasb/1 -> Terminator3/1
  ddr2_casb/1 -> Terminator7/1
  ddr2_web/1 -> Terminator8/1
  ddr2_dqs_o/1 -> Terminator11/1
  ddr2_csb/1 -> Terminator12/1
  ddr2_cke/1 -> Terminator13/1
  ddr2_dqs_i/1 -> Black Box/9
  ddr2_clk90/1 -> Black Box/10
  ddr2_clk180/1 -> Black Box/11
  ddr2_clk270/1 -> Black Box/12
  adlocb_in/1 -> Black Box/14
  ddr2_rst/1 -> Black Box/13

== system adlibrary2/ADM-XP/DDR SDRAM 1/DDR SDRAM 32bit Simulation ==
  cache_data_in : Inport  Port=1  LatchInput=off
  cache_addr : Inport  Port=2  LatchInput=off
  cache_write : Inport  Port=3  LatchInput=off
  ddr_page : Inport  Port=4  LatchInput=off
  ddr_addr : Inport  Port=5  LatchInput=off
  ddr_read : Inport  Port=6  LatchInput=off
  ddr_write : Inport  Port=7  LatchInput=off
  Disregard Subsystem : xbsIndex_r3/Disregard Subsystem  Tag=discardX
  S-Function : S-Function  FunctionName=ddr32  Parameters=memsize,1
  Subsystem : Subsystem  AncestorBlock=adlibrary2/ADM-XRC-II/XRM DDR SDRAM /DDR SDRAM 64bit Simulation/Subsystem
  Terminator13 : Terminator
  gi{0..6} (7 alike) : xbsIndex_r3/Gateway Out  output_type=Double  nbits=8  bin_pt=6  arith_type=Boolean  quantization=Truncate  overflow=Wrap  hdl_port=off  timing_constraint=None  locs_specified=off  LOCs={}  needs_fixed_name=off  show_param=off
  cache_data_out : Outport
  ddr_busy : Outport  Port=2
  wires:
  S-Function/3 -> Terminator13/1
  Subsystem/2(Out2) -> ddr_busy/1
  Subsystem/1(Out1) -> cache_data_out/1
  S-Function/1 -> Subsystem/1(In1)
  S-Function/2 -> Subsystem/2(In2)
  gi6/1 -> S-Function/7
  gi5/1 -> S-Function/6
  gi4/1 -> S-Function/5
  gi3/1 -> S-Function/4
  gi2/1 -> S-Function/3
  gi1/1 -> S-Function/2
  gi0/1 -> S-Function/1
  ddr_write/1 -> gi6/1
  ddr_read/1 -> gi5/1
  ddr_addr/1 -> gi4/1
  ddr_page/1 -> gi3/1
  cache_write/1 -> gi2/1
  cache_addr/1 -> gi1/1
  cache_data_in/1 -> gi0/1

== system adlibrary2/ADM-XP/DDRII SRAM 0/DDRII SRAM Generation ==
  d : Inport  Port=1  LatchInput=off
  a : Inport  Port=2  LatchInput=off
  w : Inport  Port=3  LatchInput=off
  r : Inport  Port=4  LatchInput=off
  be : Inport  Port=5  LatchInput=off
  adlocb_in : Inport  Port=6  LatchInput=off
  Black Box : S-Function  FunctionName=xlblackbox2  Parameters=sfcn_mwsv__  mask(Xilinx Blackbox Block){init_code=d2sram_config, sim_method=Inactive, engine_block=, show_param=off, xl_area=[0, 0, 0, 0, 0, 0, 0], xl_use_area=off, adlocb_devid=0}
      mask prompts: init_code "Block Configuration M-Function"; sim_method "Simulation Mode"; engine_block "HDL Co-Simulator To Use  (specify helper block by name)"; show_param "---------------------- Show Implementation Parameters -----------------------------------------------------------------------------------"; xl_area "FPGA Area [Slices, FFs, BRAMs, LUTs, IOBs, Emb. Mults, TBUFs]"; xl_use_area "Use Area Above For Estimation"; adlocb_devid "ADLOCB DEV ID"
      mask help: Incorporates black box HDL and simulation model into a System Generator design. You must supply a Black Box with certain information about the HDL component you would like to bring into System Generator. This information is provided through a Matlab function. When "Simulation Mode" is set to "Inactive," you will typically want to provide a separate simulation model by using a Simulation Multiplexer. When "Simulation Mode" is set to "Use HDL Co-Simulation", you must include a ModelSim block in the design.
      mask init:
      | [designRoot, family, part, speed, package, simulinkPeriod, sysclkPeriod, dbl_ovrd, trimVbit] = xlSysgenSettings(gcb,0,0);
      | 
      | [bg,fg] = xlcmap('XBlock');
      | iPos = get_param(gcb,'Position');
      | iWidth=iPos(3)-iPos(1); iHeight=iPos(4)-iPos(2);
      | iCx=iWidth/2;
      | iCy=iHeight/2;
      | [logoX, logoY] = xlogo(iPos);
      | zstr='z'; zpstr='-1';
      | zstrx = iCx-3; if (zstrx<16) zstr='';zpstr=''; end
      | zstry = iCy;
      | 
      | precision0 = 1;
      | latency = 0;
      | dblOvrd = 0;
      | 
      | mdlPath = xlGetMdlDir(bdroot);
      | 
      | refBlk = get_param(gcb,'referenceBlock');
      | if (isempty(refBlk) | strncmp(refBlk,'xbsIndex',8))
      | 	srcPath = mdlPath;
      | else
      | 	srcPath = xlPathToReference;
      | 	if (isempty(srcPath))
      | 		srcPath = mdlPath;
      | 	end
      | end
      | 
      | if (sim_method==2)
      | 	validEngineBlock = 0;
      | 	try
      | 	  engineBlock = xlBlockNameRelPath(get_param(gcb,'Parent'),engine_block);
      | 	catch
      | 	  engineBlock = '//';
      | 	end
      | 	try 
      | 	  engineWorkDir = get_param(engineBlock,'dir');
      | 	  validEngineBlock = 1;
      | 	catch
      | 	end
      | end
      | 
      | % just pass everything to s-function
      | sfcn_mwsv__ = get_param(gcb, 'MaskWSVariables');
      | 
      | plabel = xlbbPortLabelStruct(gcb,init_code,mdlPath);
  Constant : Constant  Value=0
  Convert : xbsIndex_r3/Convert  arith_type=Unsigned  n_bits=66  bin_pt=0  quantization=Truncate  overflow=Wrap  latency=0  explicit_period=on  period=1  dbl_ovrd=off  show_param=off  inserted_by_tool=off  pipeline=off
  Terminator{,1..3} (4 alike) : Terminator
  r0_clk180 : xbsIndex_r3/Gateway In  arith_type=Boolean  n_bits=1  bin_pt=0  quantization=Truncate  overflow=Wrap  period=1  timing_constraint=None  locs_specified=off  LOCs={}  needs_fixed_name=off  dbl_ovrd=off  show_param=off
  r0_clk270 : xbsIndex_r3/Gateway In  arith_type=Boolean  n_bits=1  bin_pt=0  quantization=Truncate  overflow=Wrap  period=1  timing_constraint=None  locs_specified=off  LOCs={}  needs_fixed_name=off  dbl_ovrd=off  show_param=off
  r0_clk90 : xbsIndex_r3/Gateway In  arith_type=Boolean  n_bits=1  bin_pt=0  quantization=Truncate  overflow=Wrap  period=1  timing_constraint=None  locs_specified=off  LOCs={}  needs_fixed_name=off  dbl_ovrd=off  show_param=off
  r0_rst : xbsIndex_r3/Gateway In  arith_type=Boolean  n_bits=1  bin_pt=0  quantization=Truncate  overflow=Wrap  period=1  timing_constraint=None  locs_specified=off  LOCs={}  needs_fixed_name=off  dbl_ovrd=off  show_param=off
  ra0 : xbsIndex_r3/Gateway Out  output_type=Double  nbits=8  bin_pt=6  arith_type=Boolean  quantization=Truncate  overflow=Wrap  hdl_port=on  timing_constraint=None  locs_specified=off  LOCs={}  needs_fixed_name=off  show_param=off
  rc0 : xbsIndex_r3/Gateway Out  output_type=Double  nbits=8  bin_pt=6  arith_type=Boolean  quantization=Truncate  overflow=Wrap  hdl_port=on  timing_constraint=None  locs_specified=off  LOCs={}  needs_fixed_name=off  show_param=off
  rd0_i : xbsIndex_r3/Gateway In  arith_type=Unsigned  n_bits=32  bin_pt=0  quantization=Truncate  overflow=Wrap  period=1  timing_constraint=None  locs_specified=off  LOCs={}  needs_fixed_name=off  dbl_ovrd=off  show_param=off
  rd0_o : xbsIndex_r3/Gateway Out  output_type=Double  nbits=8  bin_pt=6  arith_type=Boolean  quantization=Truncate  overflow=Wrap  hdl_port=on  timing_constraint=None  locs_specified=off  LOCs={}  needs_fixed_name=off  show_param=off
  rd0_t : xbsIndex_r3/Gateway Out  output_type=Double  nbits=8  bin_pt=6  arith_type=Boolean  quantization=Truncate  overflow=Wrap  hdl_port=on  timing_constraint=None  locs_specified=off  LOCs={}  needs_fixed_name=off  show_param=off
  q : Outport
  qv : Outport  Port=2
  adlocb_out : Outport  Port=3
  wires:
  rc0/1 -> Terminator3/1
  ra0/1 -> Terminator2/1
  rd0_t/1 -> Terminator1/1
  rd0_o/1 -> Terminator/1
  Constant/1 -> rd0_i/1, r0_rst/1, r0_clk270/1, r0_clk180/1, r0_clk90/1
  be/1 -> Black Box/7
  d/1 -> Black Box/6
  a/1 -> Black Box/5
  w/1 -> Black Box/9
  r/1 -> Black Box/8
  Black Box/4 -> rd0_t/1
  Black Box/3 -> rd0_o/1
  Black Box/2 -> rc0/1
  Black Box/1 -> ra0/1
  Black Box/5 -> q/1
  r0_rst/1 -> Black Box/10
  r0_clk270/1 -> Black Box/4
  r0_clk180/1 -> Black Box/3
  r0_clk90/1 -> Black Box/2
  rd0_i/1 -> Black Box/1
  Black Box/6 -> qv/1
  Convert/1 -> adlocb_out/1
  adlocb_in/1 -> Black Box/11
  Black Box/7 -> Convert/1

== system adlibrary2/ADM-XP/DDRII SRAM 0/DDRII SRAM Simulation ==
  d : Inport  Port=1  LatchInput=off
  a : Inport  Port=2  LatchInput=off
  w : Inport  Port=3  LatchInput=off
  r : Inport  Port=4  LatchInput=off
  be : Inport  Port=5  LatchInput=off
  Concat : xbsIndex_r3/Concat  num_inputs=2  explicit_period=off  period=1  dbl_ovrd=off
  Disregard Subsystem : xbsIndex_r3/Disregard Subsystem  Tag=discardX
  Gateway In1 : xbsIndex_r3/Gateway In  arith_type=Unsigned  n_bits=32  bin_pt=0  quantization=Truncate  overflow=Wrap  period=1  timing_constraint=None  locs_specified=off  LOCs={}  needs_fixed_name=off  dbl_ovrd=on  show_param=off
  Gateway In6 : xbsIndex_r3/Gateway In  arith_type=Boolean  n_bits=1  bin_pt=0  quantization=Truncate  overflow=Wrap  period=1  timing_constraint=None  locs_specified=off  LOCs={}  needs_fixed_name=off  dbl_ovrd=on  show_param=off
  Gateway In7 : xbsIndex_r3/Gateway In  arith_type=Unsigned  n_bits=32  bin_pt=0  quantization=Truncate  overflow=Wrap  period=1  timing_constraint=None  locs_specified=off  LOCs={}  needs_fixed_name=off  dbl_ovrd=on  show_param=off
  Gateway Out{,1..5} (6 alike) : xbsIndex_r3/Gateway Out  output_type=Double  nbits=8  bin_pt=6  arith_type=Boolean  quantization=Truncate  overflow=Wrap  hdl_port=off  timing_constraint=None  locs_specified=off  LOCs={}  needs_fixed_name=off  show_param=off
  S-Function : S-Function  FunctionName=d2sram  Parameters=0
  Slice : xbsIndex_r3/Slice  mode=Lower Bit Location + Width  nbits=32  bit1=0  base1=MSB of Input  bit0=0  base0=LSB of Input  boolean_output=off  explicit_period=off  period=1  dbl_ovrd=off
  Slice1 : xbsIndex_r3/Slice  mode=Lower Bit Location + Width  nbits=32  bit1=0  base1=MSB of Input  bit0=32  base0=LSB of Input  boolean_output=off  explicit_period=off  period=1  dbl_ovrd=off
  q : Outport
  qv : Outport  Port=2
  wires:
  Concat/1 -> q/1
  Gateway In1/1 -> Concat/2
  Gateway In7/1 -> Concat/1
  d/1 -> Slice/1, Slice1/1
  Slice/1 -> Gateway Out1/1
  Slice1/1 -> Gateway Out/1
  Gateway Out5/1 -> S-Function/6
  be/1 -> Gateway Out5/1
  S-Function/3 -> Gateway In6/1
  Gateway In6/1 -> qv/1
  S-Function/2 -> Gateway In1/1
  Gateway Out4/1 -> S-Function/5
  r/1 -> Gateway Out4/1
  Gateway Out3/1 -> S-Function/4
  Gateway Out2/1 -> S-Function/3
  Gateway Out1/1 -> S-Function/2
  Gateway Out/1 -> S-Function/1
  S-Function/1 -> Gateway In7/1
  w/1 -> Gateway Out3/1
  a/1 -> Gateway Out2/1
